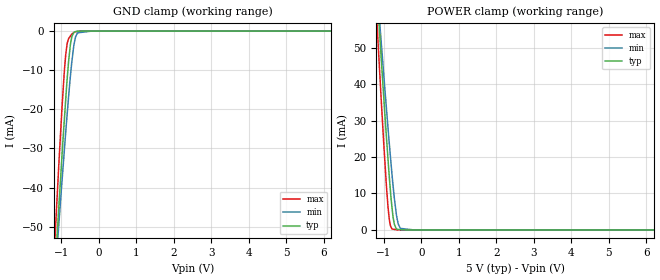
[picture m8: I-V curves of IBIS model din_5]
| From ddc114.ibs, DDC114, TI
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|   din_5 Model
[Model]   din_5
Model_type   Input
Vinl = 1
Vinh = 4
|   typ   min   max
|   (nom PVT)   (fast PVT)   (slow PVT)
|C_comp from frequency sweep method (F=55.6MHz)
|Average
|C_comp   1.527e-12   1.454e-12   1.600e-12
|C_comp from LC tank measurement(L=1nH)
|Average
|Resonant Frequency(Hz)   9.540e+09   9.590e+09   9.410e+09
C_comp   2.786e-13   2.757e-13   2.863e-13
| Where nom  PVT is Nominal Process, 5V, 27C
|   Fast PVT is Strong Process,  5.25V, -40C
|   Slow PVT is Weak Process,   4.75V, 87C
[Model Spec]
|Subparameter   typ   min   max
Vinl   1.0   0.95   1.05
Vinh   4.0   3.8   4.2
[Voltage Range]   5   4.75   5.25
|Ambient Temperature   25   85   -40
|Junction Temperature
[Temperature Range]   27   87   -40
[Power Clamp Reference]   5   4.75   5.25
[GND Clamp Reference]   0   0   0
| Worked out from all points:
|   GND clamp passes 1 mA (typ) near -0.70 V on its own axis
|   POWER clamp passes 1 mA (typ) near -0.70 V on its own axis
[GND Clamp]
|   Voltage   I(typ)   I(min)   I(max)
-5V       -715.8mA   -603.9mA   -808.2mA
-1.306V   -83.7mA    -81.6mA    -78.44mA
-1.088V   -48.25mA   -52.17mA   -38.02mA
-1.08V    -47.01mA   -51.16mA   -36.58mA
-981.8mV  -31.82mA   -38.33mA   -19.58mA
-882mV    -17.36mA   -25.78mA   -5.964mA
-840mV    -11.73mA   -20.74mA   -3.022mA
-760mV    -3.594mA   -11.75mA   -1.288mA
-640mV    -182.1uA   -2.386mA   -207.2uA
-570mV    -27.17uA   -451.4uA   -113.3uA
-190mV    0A         0A         -1.42uA
10V       0A         0A         0A
[POWER Clamp]
|   Voltage   I(typ)   I(min)   I(max)
-5V       724.8mA    612.6mA    817.4mA
-1.306V   85.76mA    83.73mA    80.17mA
-1.088V   49.89mA    53.93mA    39.05mA
-997.5mV  35.7mA     41.94mA    22.95mA
-887.2mV  19.24mA    27.84mA    6.217mA
-850.5mV  14.07mA    23.27mA    2.636mA
-782.3mV  6.226mA    15.25mA    273uA
-720mV    1.601mA    8.776mA    153.5uA
-660.3mV  297.8uA    3.884mA    38.8uA
-617.5mV  138.1uA    1.694mA    852.1nA
-560.5mV  99.23uA    436.3uA    773.5nA
10V       0A         0A         0A
